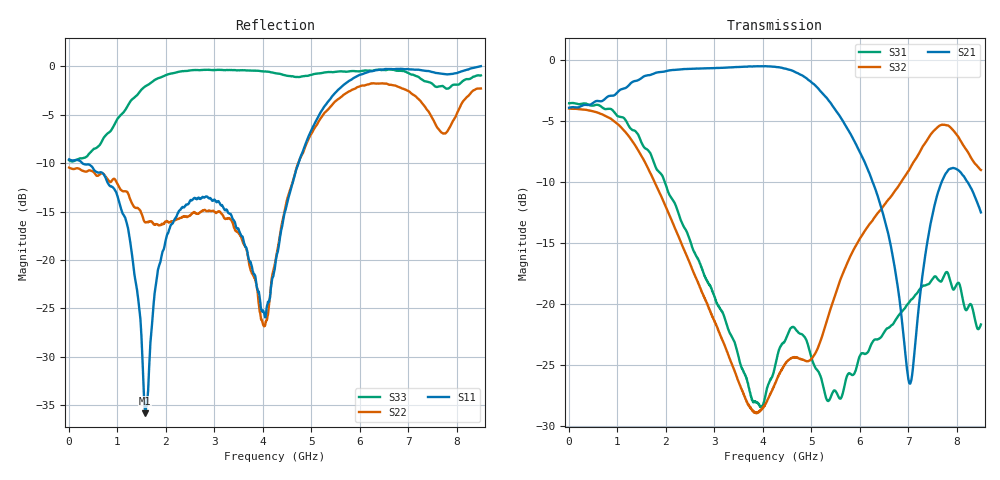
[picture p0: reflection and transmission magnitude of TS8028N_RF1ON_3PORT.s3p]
!Created with skrf (http://scikit-rf.org).
# GHz S RI R 50.0
!freq ReS11 ImS11 ReS12 ImS12 ReS13 ImS13
! ReS21 ImS21 ReS22 ImS22 ReS23 ImS23
! ReS31 ImS31 ReS32 ImS32 ReS33 ImS33
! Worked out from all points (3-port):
!   1601 points, 10 MHz to 8.5 GHz, reference 50 ohm
!   strongest paths, dB at 10 MHz, 2.132 GHz, 4.255 GHz, 6.378 GHz, 8.5 GHz:
!     S21: -3.9, -0.8, -0.5, -11.2, -12.5
!     S32: -4.0, -13.2, -26.5, -12.5, -9.0
!     S31: -3.5, -11.4, -25.1, -22.9, -21.7
!   lowest |S11| = -35.9 dB at 1.581 GHz (marker M1), VSWR 1.03, Z = 51.2 + j1.1 ohm
!   |S11| at or under -10 dB: 283.4 MHz to 4.74 GHz (4.457 GHz wide, 177 % of centre)
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0.01  -0.3308 0.00673  0.6382 0.00215  0.6654 -0.00425
      0.638 0.00205  -0.3001 0.00732  0.6329 -0.00573
      0.6653 -0.00437  0.6331 -0.00581  -0.3273 0.0137
1.182681  -0.1241 0.1008  0.7516 -0.1678  0.1455 -0.5452
          0.7514 -0.1676  -0.1638 0.156  0.0718 -0.4983
          0.1459 -0.5453  0.0721 -0.4987  0.5492 0.2522
1.58065  0.012 0.0107  0.7921 -0.3406  -0.0671 -0.4292
         0.7917 -0.3408  -0.119 0.1012  -0.1283 -0.3564
         -0.0667 -0.4292  -0.1285 -0.3567  0.768 -0.1824
2.312912  0.1071 -0.1479  0.6425 -0.6538  -0.1578 -0.1546
          0.6426 -0.6538  -0.1313 0.1  -0.1508 -0.0973
          -0.1574 -0.1546  -0.151 -0.0973  0.5788 -0.7444
4.255  -0.049 0.078  -0.282 -0.8957  -0.0227 -0.0506
       -0.2832 -0.8951  -0.0821 -0.0498  0.035 0.0318
       -0.0229 -0.0506  0.0349 0.0318  -0.7944 -0.473
4.981956  0.1148 0.4405  -0.6435 -0.505  -0.058 0.0242
          -0.6445 -0.5045  -0.4401 -0.00157  0.0589 -0.00383
          -0.058 0.0243  0.0588 -0.00377  -0.0245 0.9028
6.467706  0.6349 0.7258  -0.2239 0.0843  0.0566 -0.0481
          -0.2244 0.0846  0.1532 0.8039  0.1747 -0.1775
          0.0568 -0.0482  0.1746 -0.177  0.9416 0.1835
7.040781  0.667 0.6985  -0.0399 -0.0247  0.0417 -0.0938
          -0.0401 -0.0248  0.639 0.3656  0.1078 -0.345
          0.0418 -0.094  0.1083 -0.3438  0.9036 0.1402
7.645694  0.5733 0.7206  -0.1416 -0.2637  -0.0453 -0.1158
          -0.1422 -0.2625  0.02 -0.4673  -0.3077 -0.4395
          -0.0458 -0.1157  -0.3074 -0.4418  0.739 0.2744
8.5  0.4481 0.8983  -0.2349 0.0345  -0.0817 0.0107
     -0.235 0.0349  0.0206 0.7693  -0.3022 0.1859
     -0.0817 0.0108  -0.3025 0.1849  0.8125 0.3842
